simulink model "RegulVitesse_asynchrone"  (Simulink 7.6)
settings: Solver=ode15s  StartTime=0.0  StopTime=N  MaxStep=1e-3  MinStep=1e-4  RelTol=1e-4  AbsTol=1e-4
InitFcn:
  | clear all
  | close all
  | clc
  | 
  | 
  | N=5;
StopFcn:
  | close all
  | load Consigne_Vitesse.mat
  | plot(x(1,:),x(2,:),x(1,:),x(3,:))
  | title('Consigne vitesse et vitesse de rotation')
  | xlabel('temps')
  | grid
  | 
  | load freq_Is.mat
  | figure
  | plotyy(y(1,:),y(2,:), y(1,:),y(3,:))
  | title('fréquence d''alimentation et courant statorique')
  | xlabel('temps')
  | grid
libraries: powerlib x6, simulink x1

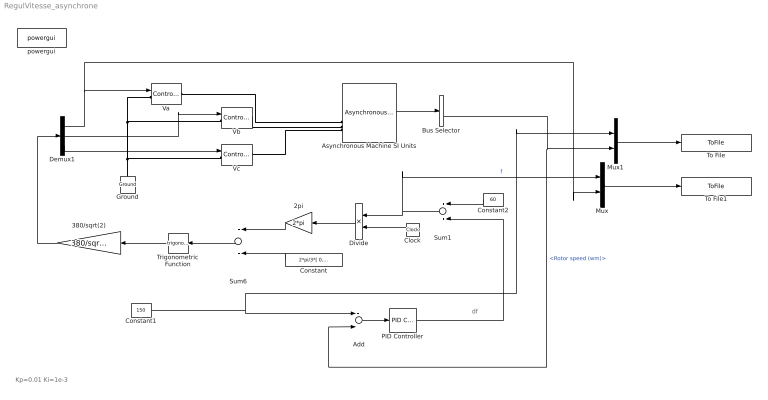
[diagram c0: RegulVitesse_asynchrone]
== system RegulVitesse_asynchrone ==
  note: df
  note: Kp=0.01 Ki=1e-3
  2pi : Gain  Gain=2*pi
  380/sqrt(2) : Gain  Gain=380/sqrt(2)
  Add : Sum  Inputs=+-
  Asynchronous Machine SI Units : powerlib/Machines/Asynchronous Machine SI Units  DialogController=POWERSYS.PowerSysDialog  SystemSampleTime=-1  PresetModel=No  MechanicalLoad=Torque Tm  ShowDetailedParameters=on  RotorType=Squirrel-cage  ReferenceFrame=Stationary  NominalParameters=[ 3800, 380, 60 ]  Stator=[ 0.029 0.226/377]  Rotor=[ 0.022 0.226/377]  Cage1=[ 0.022 0.226/377]  Cage2=[ 0.022 0.226/377]  Lm=13.04/377  Mechanical="[ 63.87 0  2 ]"  PolePairs=2  InitialConditions=[1 0 0 0 0 0 0 0]  Units=SI  LoadFlowParameters=1492000  SimulateSaturation=off  Saturation=[14.03593122, 27.81365428, 53.79336849, 72.68890987, 97.98006896, 148.6815601, 215.7428561, 302.9841135, 428.7778367 ; 230, 322, 414, 460, 506, 552, 598, 644, 690]  TsPowergui=0  TsBlock=-1  IterativeModel=Forward Euler
  Bus Selector : BusSelector  OutputSignals=Stator measurements.Stator current is_a (A),Mechanical.Rotor speed (wm)
  Clock : Clock
  Constant : Constant  Value=2*pi/3*[ 0,-1,1 ]
  Constant1 : Constant  Value=150
  Constant2 : Constant  Value=60
  Demux1 : Demux  Outputs=3
  Divide : Product  Inputs=**
  Ground : powerlib/Elements/Ground  DialogController=POWERSYS.PowerSysDialog  PhysicalDomain=powersysdomain  SubClassName=unknown  LeftPortType=p1  RightPortType=p1  LConnTagsString=a
  Mux : Mux  Inputs=2
  Mux1 : Mux  Inputs=2
  PID Controller : simulink/Continuous/PID Controller  DialogController=pidpack.PIDConfig.pidDDGCreate  DialogControllerArgs=DataTag0  SystemSampleTime=-1  Controller=PID  TimeDomain=Continuous-time  SampleTime=1  IntegratorMethod=Forward Euler  FilterMethod=Forward Euler  Form=Parallel  P=0.01  I=1e-3  D=0  N=100  InitialConditionSource=internal  InitialConditionForIntegrator=0  InitialConditionForFilter=0  ExternalReset=none  LimitOutput=off  UpperSaturationLimit=inf  LowerSaturationLimit=-inf  LinearizeAsGain=off  AntiWindupMode=none  Kb=1  TrackingMode=off  Kt=1  PParamMin=[]  PParamMax=[]  IParamMin=[]  IParamMax=[]  DParamMin=[]  DParamMax=[]  NParamMin=[]  NParamMax=[]  KbParamMin=[]  KbParamMax=[]  KtParamMin=[]  KtParamMax=[]  POutMin=[]  POutMax=[]  IOutMin=[]  IOutMax=[]  DOutMin=[]  DOutMax=[]  NOutMin=[]  NOutMax=[]  KbOutMin=[]  KbOutMax=[]  KtOutMin=[]  KtOutMax=[]  IntegratorOutMin=[]  IntegratorOutMax=[]  FilterOutMin=[]  FilterOutMax=[]  SumOutMin=[]  SumOutMax=[]  SumI1OutMin=[]  SumI1OutMax=[]  SumI2OutMin=[]  SumI2OutMax=[]  SumI3OutMin=[]  SumI3OutMax=[]  SumDOutMin=[]  SumDOutMax=[]  SaturationOutMin=[]  SaturationOutMax=[]  IntegratorContinuousStateAttributes=''  IntegratorStateMustResolveToSignalObject=off  IntegratorRTWStateStorageClass=Auto  FilterContinuousStateAttributes=''  FilterStateMustResolveToSignalObject=off  FilterRTWStateStorageClass=Auto
  Sum1 : Sum
  Sum6 : Sum
  To File : ToFile  Filename=Consigne_Vitesse  MatrixName=x
  To File1 : ToFile  Filename=freq_Is  MatrixName=y
  Trigonometric Function : Trigonometry
  Va : powerlib/Electrical Sources/Controlled Voltage Source  Description=source block  DialogController=POWERSYS.PowerSysDialog  SystemSampleTime=-1  Initialize=on  Source_Type=AC  Amplitude=0  Phase=0  Frequency=0  Measurements=None
  Vb : powerlib/Electrical Sources/Controlled Voltage Source  Description=source block  DialogController=POWERSYS.PowerSysDialog  SystemSampleTime=-1  Initialize=on  Source_Type=AC  Amplitude=0  Phase=0  Frequency=0  Measurements=None
  Vc : powerlib/Electrical Sources/Controlled Voltage Source  Description=source block  DialogController=POWERSYS.PowerSysDialog  SystemSampleTime=-1  Initialize=on  Source_Type=AC  Amplitude=0  Phase=0  Frequency=0  Measurements=None
  powergui : powerlib/powergui  Priority=2  SystemSampleTime=-1  SimulationMode=Continuous  SampleTime=1e-5  frequency=60  SPID=off  DisableSnubberDevices=off  DisableRonSwitches=off  DisableVfSwitches=off  SwTol=0  Interpol=off  frequencyindice=60  echomessages=off  HookPort=off  DisplayEquations=off  FunctionMessages=off  EnableUseOfTLC=off  x0status=blocks  RestoreLinks=warning  ResistiveCurrentMeasurement=off  Frange=[0:2:500]  Ylog=off  Xlog=on  ShowGrid=off  save=off  variable=ZData  ZoomFFT=on  StartTime=0.0  cycles=1  DisplayStyle=1  fundamental=60  FreqAxis=off  MaxFrequency=1000  frequencyindicesteady=1  RmsSteady=1  display=off  Ts=0  methode=off
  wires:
  Asynchronous Machine SI Units/1 -> Bus Selector/1
  Mux/1 -> To File1/1
  Bus Selector/2 -> Mux1/2, Add/2  "<Rotor speed (wm)>"
  Add/1 -> PID Controller/1
  PID Controller/1 -> Sum1/2
  Constant1/1 -> Add/1, Mux1/1
  2pi/1 -> Sum6/1
  Constant/1 -> Sum6/2
  Trigonometric Function/1 -> 380/sqrt(2)/1
  Demux1/1 -> Va/1, Mux/2
  Demux1/2 -> Vb/1
  Demux1/3 -> Vc/1
  Clock/1 -> Divide/2
  Divide/1 -> 2pi/1
  380/sqrt(2)/1 -> Demux1/1
  Sum1/1 -> Divide/1, Mux/1  "f"
  Constant2/1 -> Sum1/1
  Mux1/1 -> To File/1
  Sum6/1 -> Trigonometric Function/1
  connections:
  Vb/RConn1 -- Asynchronous Machine SI Units/LConn2
  Vc/RConn1 -- Asynchronous Machine SI Units/LConn3
  Ground/LConn1 -- Vc/LConn1 -- Va/LConn1 -- Vb/LConn1
  Va/RConn1 -- Asynchronous Machine SI Units/LConn1
